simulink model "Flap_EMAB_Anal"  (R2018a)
settings: Solver=ode45  StartTime=0.0  StopTime=1  RelTol=1e-3  EnableMultiTasking=on
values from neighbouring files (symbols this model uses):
  Be = 25    [init.m]
  Ja = 2.0e-4    (= 0.0002)    [init.m]
  Je = 2.2    [init.m]
  Jm = 5.0e-5    (= 5e-05)    [init.m]
  Kdmp = 0.001    [init.m]
  Keff = 0.85    [init.m]
  Kgs = 400.0    (= 400)    [init.m]
  Ki = 5.0    (= 5)    [init.m]
  Kl = 12/Kli    (= 1800000)    [init.m]
  Kmfr = 0.03    [init.m]
  Kp = 140    [init.m]
  Krfb = 0.0005    [init.m]
  Kt = 12/Kti    (= 1674418.60465)    [init.m]
  Kv = 260    [init.m]
  Ngear = 10.2    [init.m]
  Nscrew = 0.0026    [init.m]
  R = 0.287    [init.m]    (also in lqr_des.m = diag(R))
  Wmb = 1500    [init.m]

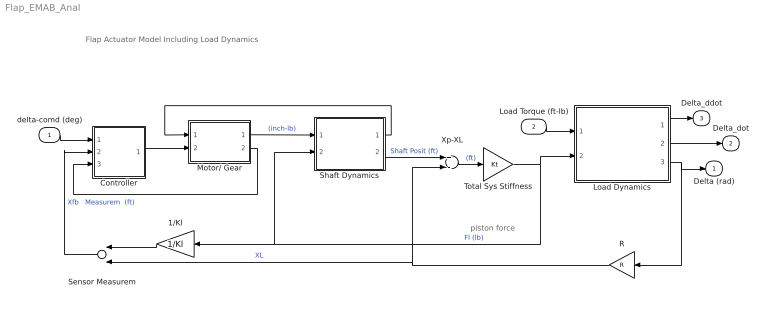
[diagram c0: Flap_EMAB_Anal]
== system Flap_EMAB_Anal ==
  note: piston force
  note: Flap Actuator Model Including Load Dynamics
  delta-comd (deg) : Inport
  Load Torque (ft-lb) : Inport  Port=2
  1/Kl : Gain  Gain=1/Kl
  Controller : Subsystem
  Load Dynamics : Subsystem
  Motor/ Gear : Subsystem
  R : Gain  Gain=R
  Sensor Measurem : Sum
  Shaft Dynamics : Subsystem
  Total Sys Stiffness : Gain  Gain=Kt
  Xp-XL : Sum  Inputs=+-
  Delta (rad) : Outport
  Delta_dot : Outport  Port=2
  Delta_ddot : Outport  Port=3
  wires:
  Shaft Dynamics/2(Xp) -> Xp-XL/1  "Shaft Posit (ft)"
  Xp-XL/1 -> Total Sys Stiffness/1  "(ft)"
  Total Sys Stiffness/1 -> Load Dynamics/2(FL), Shaft Dynamics/2(FL), 1/Kl/1  "Fl (lb)"
  1/Kl/1 -> Sensor Measurem/1
  Controller/1(V) -> Motor/ Gear/2(Vin)
  Motor/ Gear/1(Tm) -> Shaft Dynamics/1(Tq-mot)  "(inch-lb)"
  Load Dynamics/1(Del_ddot) -> Delta_ddot/1
  Load Dynamics/3(Delta (rad)) -> Delta (rad)/1, R/1
  Load Dynamics/2(Delta_dot) -> Delta_dot/1
  Sensor Measurem/1 -> Controller/2(Xp-fb)  "Xfb   Measurem  (ft)"
  delta-comd (deg)/1 -> Controller/1(delt-cmd)
  Shaft Dynamics/1(Xp-dot) -> Motor/ Gear/1(Xp-dot)
  R/1 -> Sensor Measurem/2, Xp-XL/2  "XL"
  Motor/ Gear/2(mr) -> Controller/3(rotor)
  Load Torque (ft-lb)/1 -> Load Dynamics/1(Load Torque)

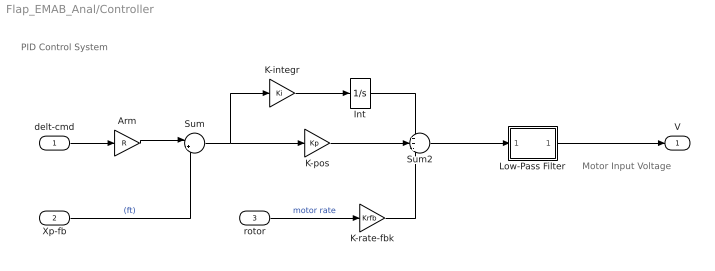
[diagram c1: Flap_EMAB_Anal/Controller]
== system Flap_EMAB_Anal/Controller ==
  note: PID Control System
  note: Motor Input Voltage
  delt-cmd : Inport
  Xp-fb : Inport  Port=2
  rotor : Inport  Port=3
  Arm : Gain  Gain=R
  Int : Integrator  UpperSaturationLimit=1  LowerSaturationLimit=-1
  K-integr : Gain  Gain=Ki
  K-pos : Gain  Gain=Kp
  K-rate-fbk : Gain  Gain=Krfb
  Low-Pass Filter : Subsystem
  Sum : Sum  Inputs=|+-
  Sum2 : Sum  Inputs=++-
  V : Outport
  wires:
  delt-cmd/1 -> Arm/1
  Xp-fb/1 -> Sum/2  "(ft)"
  Sum/1 -> K-pos/1, K-integr/1
  rotor/1 -> K-rate-fbk/1  "motor rate"
  K-pos/1 -> Sum2/2
  K-integr/1 -> Int/1
  Int/1 -> Sum2/1
  K-rate-fbk/1 -> Sum2/3
  Arm/1 -> Sum/1
  Sum2/1 -> Low-Pass Filter/1(in)
  Low-Pass Filter/1(ou) -> V/1

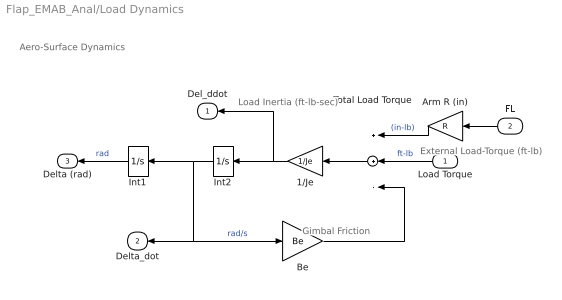
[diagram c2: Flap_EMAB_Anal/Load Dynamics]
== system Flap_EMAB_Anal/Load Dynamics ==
  note: External Load-Torque (ft-lb)
  note: Load Inertia (ft-lb-sec)
  note: Gimbal Friction
  note: Aero-Surface Dynamics
  Load Torque : Inport
  FL : Inport  Port=2
  1/Je : Gain  Gain=1/Je
  Arm R (in) : Gain  Gain=R
  Be : Gain  Gain=Be
  Int1 : Integrator
  Int2 : Integrator
  Total Load Torque : Sum  Inputs=++-
  Del_ddot : Outport
  Delta_dot : Outport  Port=2
  Delta (rad) : Outport  Port=3
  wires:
  1/Je/1 -> Del_ddot/1, Int2/1
  Int2/1 -> Delta_dot/1, Be/1, Int1/1  "rad/s"
  FL/1 -> Arm R (in)/1
  Load Torque/1 -> Total Load Torque/2  "ft-lb"
  Int1/1 -> Delta (rad)/1  "rad"
  Total Load Torque/1 -> 1/Je/1
  Be/1 -> Total Load Torque/3
  Arm R (in)/1 -> Total Load Torque/1  "(in-lb)"

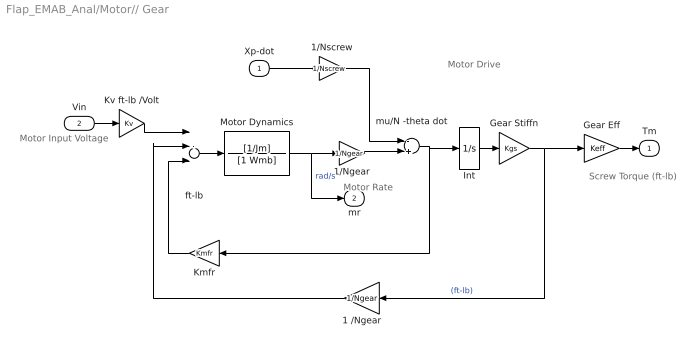
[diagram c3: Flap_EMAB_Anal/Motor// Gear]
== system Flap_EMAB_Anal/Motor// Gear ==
  note: Motor Input Voltage
  note: Motor Rate
  note: Screw Torque (ft-lb)
  note: Motor Drive
  Xp-dot : Inport
  Vin : Inport  Port=2
  1 /Ngear : Gain  Gain=1/Ngear
  1/Ngear : Gain  Gain=1/Ngear
  1/Nscrew : Gain  Gain=1/Nscrew
  Gear Eff : Gain  Gain=Keff
  Gear Stiffn : Gain  Gain=Kgs
  Int : Integrator  UpperSaturationLimit=0.4  LowerSaturationLimit=-0.4
  Kmfr : Gain  Gain=Kmfr
  Kv ft-lb /Volt : Gain  Gain=Kv
  Motor Dynamics : TransferFcn  Numerator=[1/Jm]  Denominator=[1 Wmb]
  ft-lb : Sum  Inputs=+---
  mu/N -theta dot : Sum  Inputs=-+
  Tm : Outport
  mr : Outport  Port=2
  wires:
  Int/1 -> Gear Stiffn/1
  Kmfr/1 -> ft-lb/3
  1/Nscrew/1 -> mu/N -theta dot/1
  Kv ft-lb /Volt/1 -> ft-lb/1
  Gear Eff/1 -> Tm/1
  Vin/1 -> Kv ft-lb /Volt/1
  Xp-dot/1 -> 1/Nscrew/1
  Gear Stiffn/1 -> Gear Eff/1, 1 /Ngear/1  "(ft-lb)"
  1/Ngear/1 -> mu/N -theta dot/2
  Motor Dynamics/1 -> mr/1, 1/Ngear/1  "rad/s"
  1 /Ngear/1 -> ft-lb/2
  ft-lb/1 -> Motor Dynamics/1
  mu/N -theta dot/1 -> Kmfr/1, Int/1

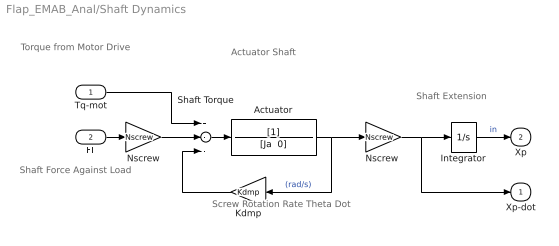
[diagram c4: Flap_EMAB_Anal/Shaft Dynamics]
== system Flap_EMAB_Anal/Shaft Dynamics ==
  note: Screw Rotation Rate Theta Dot
  note: Shaft Extension
  note: Actuator Shaft
  note: Shaft Force Against Load
  note: Torque from Motor Drive
  Tq-mot : Inport
  FL : Inport  Port=2
  Actuator : TransferFcn  Denominator="[Ja  0]"
  Integrator : Integrator
  Kdmp : Gain  Gain=Kdmp
  Nscrew : Gain  Gain=Nscrew
  "Nscrew " : Gain  Gain=Nscrew
  Shaft Torque : Sum  Inputs=+--
  Xp-dot : Outport
  Xp : Outport  Port=2
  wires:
  Kdmp/1 -> Shaft Torque/3
  "Nscrew "/1 -> Xp-dot/1, Integrator/1
  Nscrew/1 -> Shaft Torque/2
  FL/1 -> Nscrew/1
  Integrator/1 -> Xp/1  "in"
  Tq-mot/1 -> Shaft Torque/1
  Shaft Torque/1 -> Actuator/1
  Actuator/1 -> Kdmp/1, "Nscrew "/1  "(rad/s)"

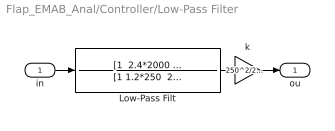
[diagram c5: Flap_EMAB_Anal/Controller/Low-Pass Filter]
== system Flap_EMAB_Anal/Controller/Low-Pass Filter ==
  in : Inport
  Low-Pass Filt : TransferFcn  Numerator="[1  2.4*2000  2000^2]"  Denominator="[1 1.2*250  250^2]"
  k : Gain  Gain=250^2/2000^2
  ou : Outport
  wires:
  k/1 -> ou/1
  in/1 -> Low-Pass Filt/1
  Low-Pass Filt/1 -> k/1
